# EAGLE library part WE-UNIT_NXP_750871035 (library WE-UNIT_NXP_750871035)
Off-Line Transformer WE-Unit NXP - Nominal input voltage: 85-265 VAC - Operating temperature: -40°C to +125 °C - Isolation voltage 4 kVAC -- Especially designed for several ICs from NXP TEA1522T -- Universal input -- Smart meters -- Dimmable 12 V LED driver -- Offline-switch mode power supplies
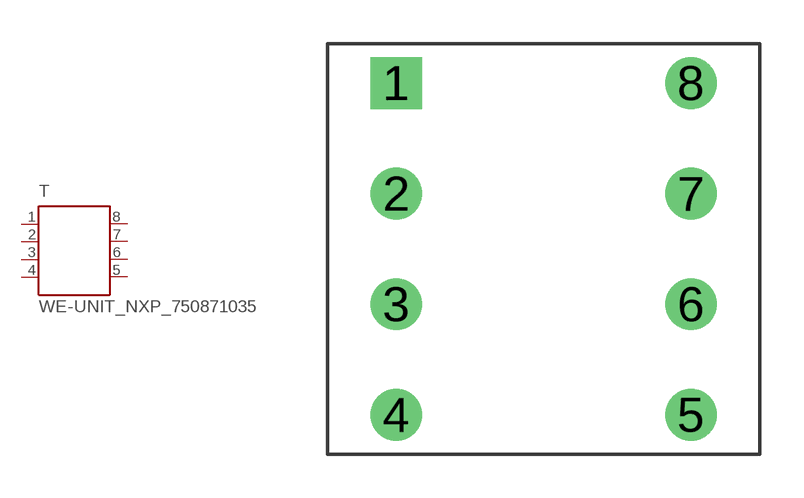
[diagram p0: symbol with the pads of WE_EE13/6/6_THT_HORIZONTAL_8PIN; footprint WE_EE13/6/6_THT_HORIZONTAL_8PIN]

Designator prefix T

## WE-UNIT_NXP_750871035 (MPN: 750871035; OC_FARNELL: 1849053; OC_NEWARK: 13T9842; PACKAGE: EE13_6_6; SUPPLIER: Würth Elektronik eiSos GmbH)  [WE_EE13/6/6_THT_HORIZONTAL_8PIN]
1  4  pas
2  3  pas
3  2  pas
4  1  pas
5  8  pas
6  7  pas
7  6  pas
8  5  pas

## Footprint WE_EE13/6/6_THT_HORIZONTAL_8PIN (pad centres in mm)
Transformer, EE13/6/6 THT Horizontal 8 Pins
drill 1.19 square: 1 -5.075,5.715
drill 1.19: 2 -5.075,1.905; 3 -5.075,-1.905; 4 -5.075,-5.715; 5 5.075,-5.715; 6 5.075,-1.905; 7 5.075,1.905; 8 5.075,5.715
